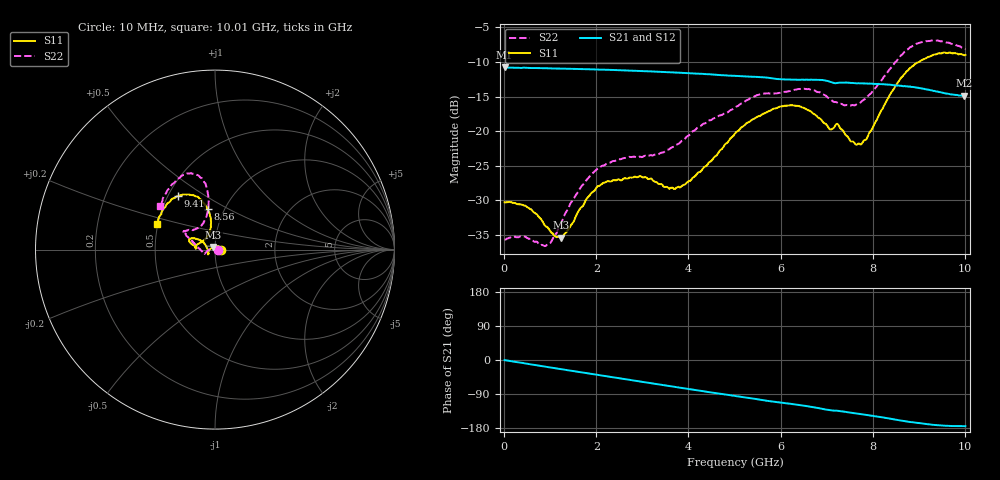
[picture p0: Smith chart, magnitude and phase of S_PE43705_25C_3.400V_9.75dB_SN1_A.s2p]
! Device ID: PE43705
! Serial: 1
! Insertion: A
! Impedance: 50 ohm
! Temp: 25C
! VDD: 3.400V
! Attenuation Step: 9.75dB
#  Hz  S  RI  R  50
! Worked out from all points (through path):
!   401 points, 10 MHz to 10.01 GHz, reference 50 ohm
!   highest |S21| = -10.79 dB at 10 MHz (marker M1); lowest = -14.9 dB at 9.985 GHz (marker M2)
!   group delay of S21, straight-line fit = 50.2 ps
!   lowest |S11| = -35.4 dB at 1.235 GHz (marker M3), VSWR 1.03, Z = 49.1 + j1.43 ohm
!   |S11| at or under -10 dB: start of sweep to 9.003 GHz
!   |S22| runs from -36.6 to -6.9 dB; largest |S21 - S12| = 0.0025
!   S11 on the Smith chart (normalised r, x): 10 MHz: 1.06, +0.00; 8.56 GHz: 0.84, +0.40; 9.41 GHz: 0.56, +0.39; 10.01 GHz: 0.49, +0.16
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1e7  0.0307 0.000179  0.2886 -0.00138  0.2889 -0.0012  0.0165 0.000239
4.85e8  0.0236 0.0159  0.2825 -0.0483  0.2827 -0.048  0.0109 0.0131
9.1e8  0.0065 0.0194  0.2709 -0.0877  0.2709 -0.0874  -0.00493 0.0141
1.235e9  -0.00886 0.0145  0.2583 -0.1156  0.2584 -0.1154  -0.0202 0.008
1.685e9  -0.0284 0.000954  0.2361 -0.1518  0.2361 -0.1518  -0.04 -0.0052
2.21e9  -0.0395 -0.0171  0.2038 -0.1885  0.204 -0.1884  -0.0543 -0.02
2.96e9  -0.0395 -0.0262  0.1479 -0.2282  0.1481 -0.2282  -0.0623 -0.0193
3.36e9  -0.036 -0.0207  0.1154 -0.2423  0.1157 -0.242  -0.0669 -0.0143
3.885e9  -0.0407 0.000204  0.0711 -0.2535  0.0713 -0.2533  -0.0855 0.00359
5.01e9  -0.0808 0.0519  -0.0211 -0.25  -0.0208 -0.2499  -0.1376 0.0567
5.985e9  -0.1371 0.0616  -0.0895 -0.22  -0.0884 -0.2201  -0.165 0.0925
6.685e9  -0.1319 0.0323  -0.132 -0.1946  -0.132 -0.1944  -0.1678 0.1042
7.06e9  -0.1025 0.0135  -0.1539 -0.1681  -0.1534 -0.1691  -0.1312 0.1111
7.335e9  -0.0977 0.0306  -0.1596 -0.1572  -0.1597 -0.1578  -0.1042 0.1171
7.71e9  -0.0537 0.0609  -0.1752 -0.1357  -0.1751 -0.1359  -0.068 0.1443
7.91e9  -0.0342 0.0888  -0.1822 -0.1237  -0.1823 -0.1251  -0.0535 0.1733
8.36e9  -0.0241 0.1785  -0.1955 -0.0935  -0.1948 -0.0943  -0.0366 0.2759
8.56e9  -0.0394 0.225  -0.1995 -0.0769  -0.1978 -0.0786  -0.0415 0.3345
8.96e9  -0.1017 0.2953  -0.1997 -0.0502  -0.1987 -0.0497  -0.1029 0.4167
9.41e9  -0.2049 0.2996  -0.1912 -0.0265  -0.1905 -0.0262  -0.1837 0.413
9.985e9  -0.3185 0.1521  -0.1793 -0.0171  -0.1803 -0.0177  -0.2985 0.2561
1.001e10  -0.3252 0.1429  -0.1801 -0.017  -0.1812 -0.0182  -0.3057 0.2455
